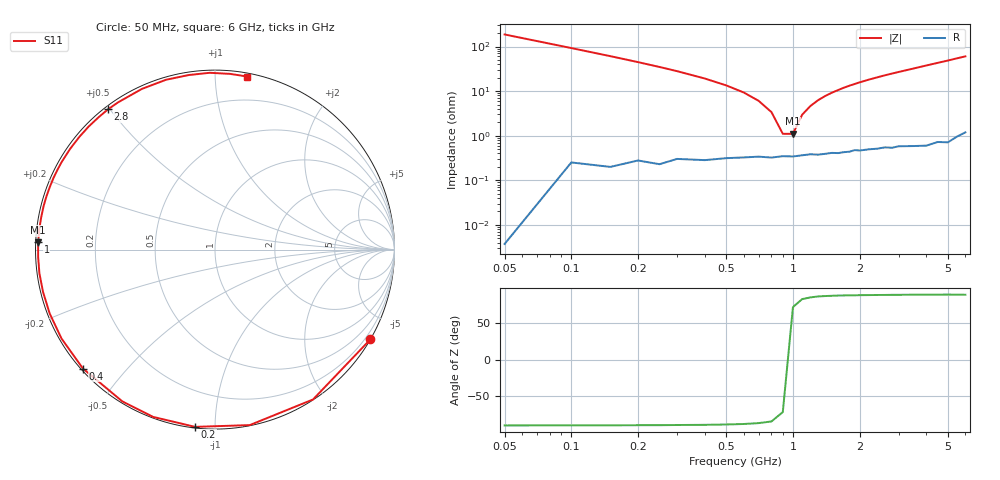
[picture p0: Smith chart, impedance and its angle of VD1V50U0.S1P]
! Infineon Technologies  Discrete & RF Semiconductors
! BBY 55-03
! Si Tuning Diode in SOD323
! VR = 1.5 V
! S-Parameters:  June  1999
# GHz  S  MA  R  50
!  f  S11
! GHz  MAG  ANG
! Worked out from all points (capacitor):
!   34 points, 50 MHz to 6 GHz, reference 50 ohm
!   read as one part to ground: C = 17 pF near 50 MHz
!   lowest |Z| = 1.1 ohm at 1 GHz (marker M1)
!   series resonance near 950 MHz, so ESL is about 1.6 nH
!   S11 on the Smith chart (normalised r, x): 50 MHz: 0.00, -3.73; 200 MHz: 0.01, -0.89; 400 MHz: 0.01, -0.38; 1 GHz: 0.01, +0.02; 2.8 GHz: 0.01, +0.50; 6 GHz: 0.02, +1.20
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0.05  1 -30.0
0.1  0.9977 -56.8
0.15  0.9968 -78.8
0.2  0.9938 -96.4
0.25  0.9938 -110.3
0.3  0.9909 -121.4
0.4  0.9902 -138.0
0.5  0.9884 -149.9
0.6  0.9875 -158.9
0.7  0.9867 -166.2
0.8  0.9872 -172.3
1  0.9864 177.6
1.1  0.9856 173.3
1.3  0.9853 165.7
1.4  0.9848 162.3
1.6  0.9845 156.1
1.8  0.9838 150.3
2  0.9832 145.1
2.2  0.9827 140.2
2.4  0.9826 135.7
2.8  0.9829 127.3
3  0.9822 123.4
3.5  0.9836 114.5
4  0.9848 106.1
4.5  0.9836 98.5
5  0.9855 91.7
5.5  0.9827 85.1
6  0.9808 79.4
